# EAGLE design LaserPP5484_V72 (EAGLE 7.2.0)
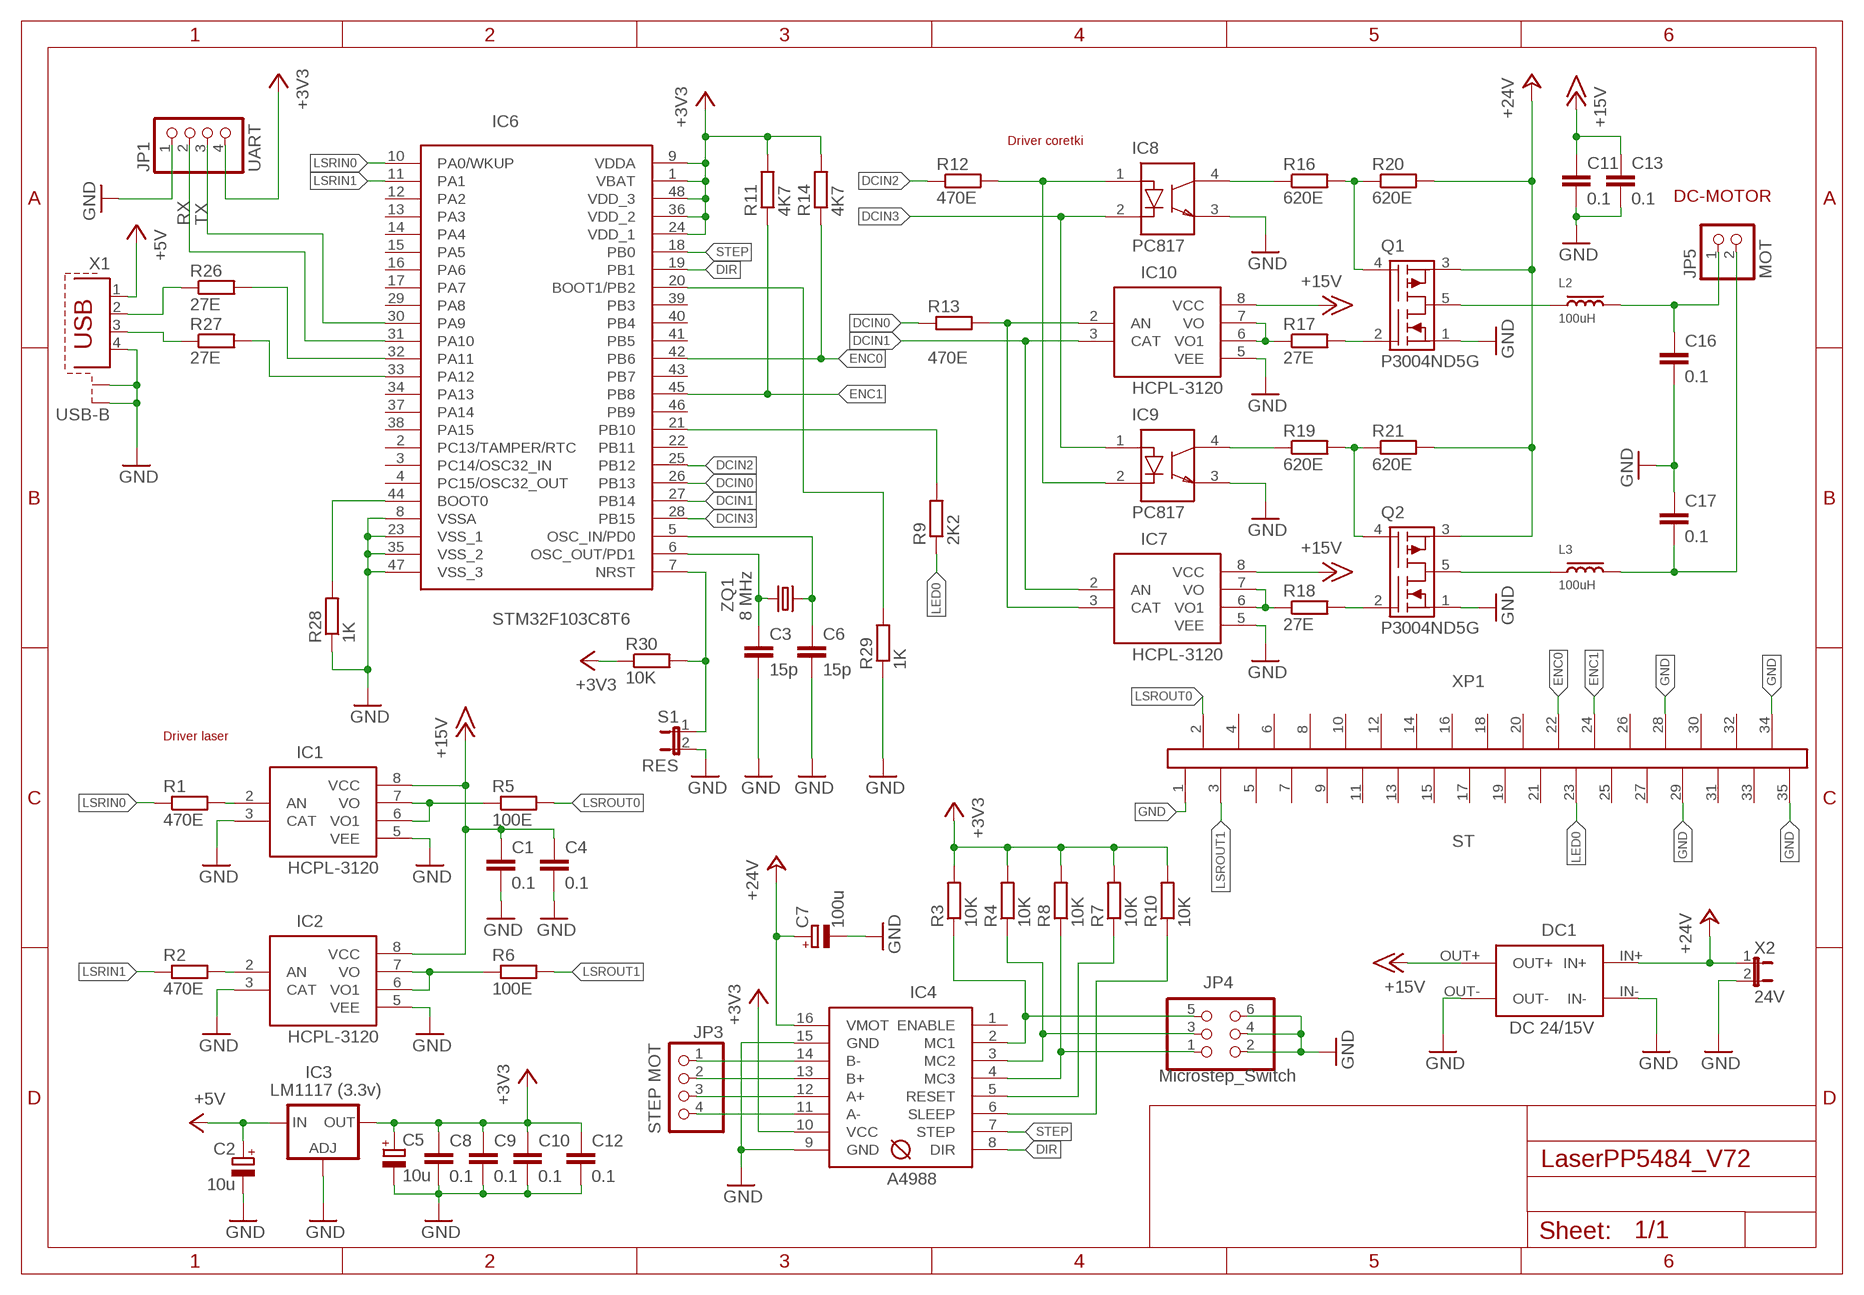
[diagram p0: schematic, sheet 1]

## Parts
C1  0.1  C-EUC0805  [C0805]
C2  10u  CPOL-EUSMCC  [SMC_C]
C3  15p  C-EUC0805  [C0805]
C4  0.1  C-EUC0805  [C0805]
C5  10u  CPOL-EUSMCA  [SMC_A]
C6  15p  C-EUC0805  [C0805]
C7  100u  CPOL-EUE2.5-7  [E2,5-7]
C8  0.1  C-EUC0805  [C0805]
C9  0.1  C-EUC0805  [C0805]
C10  0.1  C-EUC0805  [C0805]
C11  0.1  C-EUC0805  [C0805]
C12  0.1  C-EUC0805  [C0805]
C13  0.1  C-EUC0805  [C0805]
C16  0.1  C-EUC0805  [C0805]
C17  0.1  C-EUC0805  [C0805]
DC1  DC 24/15V  DC  [DC]
IC1  HCPL-3120  HCPL-3120DILSMD  [DIL08SMD]
IC2  HCPL-3120  HCPL-3120DILSMD  [DIL08SMD]
IC3  LM1117 (3.3v)  LM317MBSTT3  [SOT223]
IC4  A4988  [A4988]
IC6  STM32F103C8T6  STM32F100C4T  [LQFP48-7X7]
IC7  HCPL-3120  HCPL-3120DILSMD  [DIL08SMD]
IC8  PC817  [DIL04]
IC9  PC817  [DIL04]
IC10  HCPL-3120  HCPL-3120DILSMD  [DIL08SMD]
JP1  UART  PINHD-1X4  [1X04]
JP3  STEP MOT  PINHD-1X4  [1X04]
JP4  Microstep_Switch  PINHD-2X3  [2X03]
JP5  MOT  PINHD-1X2PW10-2-M  [PW10-2-M]
L2  100uH  L  [5_08]
L3  100uH  L  [5_08]
Q1  P3004ND5G  [TO252-51]
Q2  P3004ND5G  [TO252-51]
R1  470E  R-EU_R0805  [R0805]
R2  470E  R-EU_R0805  [R0805]
R3  10K  R-EU_R0805  [R0805]
R4  10K  R-EU_R0805  [R0805]
R5  100E  R-EU_0617/22  [0617/22]
R6  100E  R-EU_0617/22  [0617/22]
R7  10K  R-EU_R0805  [R0805]
R8  10K  R-EU_R0805  [R0805]
R9  2K2  R-EU_R0805  [R0805]
R10  10K  R-EU_R0805  [R0805]
R11  4K7  R-EU_R0805  [R0805]
R12  470E  R-EU_R0805  [R0805]
R13  470E  R-EU_R0805  [R0805]
R14  4K7  R-EU_R0805  [R0805]
R16  620E  R-EU_R0805  [R0805]
R17  27E  R-EU_R1206  [R1206]
R18  27E  R-EU_R1206  [R1206]
R19  620E  R-EU_R0805  [R0805]
R20  620E  R-EU_R0805  [R0805]
R21  620E  R-EU_R0805  [R0805]
R26  27E  R-EU_R1206  [R1206]
R27  27E  R-EU_R1206  [R1206]
R28  1K  R-EU_R0805  [R0805]
R29  1K  R-EU_R0805  [R0805]
R30  10K  R-EU_R0805  [R0805]
S1  RES  JP1E  [JP1]
X1  USB-B  PN61729-S  [PN61729-S]
X2  24V  PWL  [PWL]
XP1  ST  [ST]
ZQ1  8 MHz  CRYSTALHC49S  [HC49/S]

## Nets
+3V3: C5.+ C8.1 C9.1 C10.1 C12.1 IC3.4(OUT) IC4.10(VCC) IC6.1(VBAT) IC6.9(VDDA) IC6.24(VDD_1) IC6.36(VDD_2) IC6.48(VDD_3) JP1.4 R3.2 R4.2 R7.2 R8.2 R10.2 R11.2 R14.2 R30.1
+5V: C2.+ IC3.3(IN) X1.1
+15V: C1.1 C4.1 C11.1 C13.1 DC1.OUT+ IC1.8(VCC) IC2.8(VCC) IC7.8(VCC) IC10.8(VCC)
+24V: C7.+ DC1.IN+ IC4.16(VMOT) Q1.3(S2) Q2.3(S2) R20.2 R21.2 X2.1
DCIN0: IC6.26(PB13) R13.1
DCIN1: IC6.27(PB14) IC7.2(AN) IC10.3(CAT)
DCIN2: IC6.25(PB12) R12.1
DCIN3: IC6.28(PB15) IC8.2(K) IC9.1(A)
DIR: IC4.8(DIR) IC6.19(PB1)
ENC0: IC6.42(PB6) R14.1 XP1.22
ENC1: IC6.45(PB8) R11.1 XP1.24
GND: C1.2 C2.- C3.2 C4.2 C5.- C6.2 C7.- C8.2 C9.2 C10.2 C11.2 C12.2 C13.2 C16.2 C17.1 DC1.IN- DC1.OUT- IC1.3(CAT) IC1.5(VEE) IC2.3(CAT) IC2.5(VEE) IC3.1(ADJ) IC4.9(GND) IC4.15(GND) IC6.8(VSSA) IC6.23(VSS_1) IC6.35(VSS_2) IC6.47(VSS_3) IC7.5(VEE) IC8.3(E) IC9.3(E) IC10.5(VEE) JP1.1 JP4.2 JP4.4 JP4.6 Q1.1(S1) Q2.1(S1) R28.1 R29.1 S1.2 X1.4 X1.S1 X1.S2 X2.2 XP1.1 XP1.28 XP1.29 XP1.34 XP1.35
LED0: R9.1 XP1.23
LSRIN0: IC6.10(PA0/WKUP) R1.1
LSRIN1: IC6.11(PA1) R2.1
LSROUT0: R5.2 XP1.2
LSROUT1: R6.2 XP1.3
N$1: IC6.7(NRST) R30.2 S1.1
N$2: C3.1 IC6.6(OSC_OUT/PD1) ZQ1.1
N$3: C6.1 IC6.5(OSC_IN/PD0) ZQ1.2
N$4: R26.1 X1.2
N$5: IC6.32(PA11) R26.2
N$6: R27.1 X1.3
N$7: IC6.33(PA12) R27.2
N$8: IC4.11(A-) JP3.4
N$9: IC4.12(A+) JP3.3
N$10: IC1.2(AN) R1.2
N$11: IC4.13(B+) JP3.2
N$12: IC6.44(BOOT0) R28.2
N$14: IC2.2(AN) R2.2
N$15: IC6.21(PB10) R9.2
N$17: IC4.14(B-) JP3.1
N$18: IC4.2(MC1) JP4.5 R3.1
N$19: IC4.3(MC2) JP4.3 R4.1
N$20: IC4.4(MC3) JP4.1 R8.1
N$21: IC8.1(A) IC9.2(K) R12.2
N$22: IC8.4(C) R16.1
N$23: IC7.3(CAT) IC10.2(AN) R13.2
N$24: IC9.4(C) R19.1
N$25: IC10.6(VO1) IC10.7(VO) R17.1
N$26: IC7.6(VO1) IC7.7(VO) R18.1
N$27: Q1.2(G1) R17.2
N$28: L2.1 Q1.5(D1/D2)
N$29: Q1.4(G2) R16.2 R20.1
N$30: Q2.2(G1) R18.2
N$31: Q2.4(G2) R19.2 R21.1
N$32: L3.1 Q2.5(D1/D2)
N$33: C17.2 JP5.2 L3.2
N$34: C16.1 JP5.1 L2.2
N$35: IC4.5(RESET) R7.1
N$36: IC4.6(SLEEP) R10.1
N$39: IC1.6(VO1) IC1.7(VO) R5.1
N$41: IC2.6(VO1) IC2.7(VO) R6.1
N$48: IC6.20(BOOT1/PB2) R29.2
RX: IC6.31(PA10) JP1.2
STEP: IC4.7(STEP) IC6.18(PB0)
TX: IC6.30(PA9) JP1.3
Unconnected: IC4.1(ENABLE) IC6.2(PC13/TAMPER/RTC) IC6.3(PC14/OSC32_IN) IC6.4(PC15/OSC32_OUT) IC6.12(PA2) IC6.13(PA3) IC6.14(PA4) IC6.15(PA5) IC6.16(PA6) IC6.17(PA7) IC6.22(PB11) IC6.29(PA8) IC6.34(PA13) IC6.37(PA14) IC6.38(PA15) IC6.39(PB3) IC6.40(PB4) IC6.41(PB5) IC6.43(PB7) IC6.46(PB9) XP1.4 XP1.5 XP1.6 XP1.7 XP1.8 XP1.9 XP1.10 XP1.11 XP1.12 XP1.13 XP1.14 XP1.15 XP1.16 XP1.17 XP1.18 XP1.19 XP1.20 XP1.21 XP1.25 XP1.26 XP1.27 XP1.30 XP1.31 XP1.32 XP1.33

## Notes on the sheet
- Driver coretki
- DC-MOTOR
- Driver laser

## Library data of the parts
C1 C3 C4 C6 C8-C13 C16 C17 = rcl:C-EU: CAPACITOR, European symbol
C2 C5 C7 = rcl:CPOL-EU: POLARIZED CAPACITOR, European symbol
DC1 = LaserPP:DC
IC1 IC2 IC7 IC10 = LaserPP:HCPL-3120
IC3 = v-reg:LM317?*: 500 mA Adjustable Output Positive Voltage Regulator Source: http://www.onsemi.co.jp .. LM317M-D.PDF
IC4 = LaserPP:A4988
IC6 = Timer-stm32:STM32F100C4T
IC8 IC9 = LaserPP:PC817
JP1 JP3 = pinhead:PINHD-1X4: PIN HEADER
JP4 = LaserPP:PINHD-2X3: PIN HEADER
JP5 = BPPLS:PINHD-1X2: PIN HEADER
L2 L3 = LaserPP:L
Q1 Q2 = LaserPP:P3004ND5G
R1-R14 R16-R21 R26-R30 = rcl:R-EU_: RESISTOR, European symbol
S1 = jumper:JP1E: JUMPER
X1 = con-berg:PN61729-S: BERG USB connector
X2 = Timer-stm32:PWL
XP1 = LaserPP:ST
ZQ1 = crystal:CRYSTAL: CRYSTAL

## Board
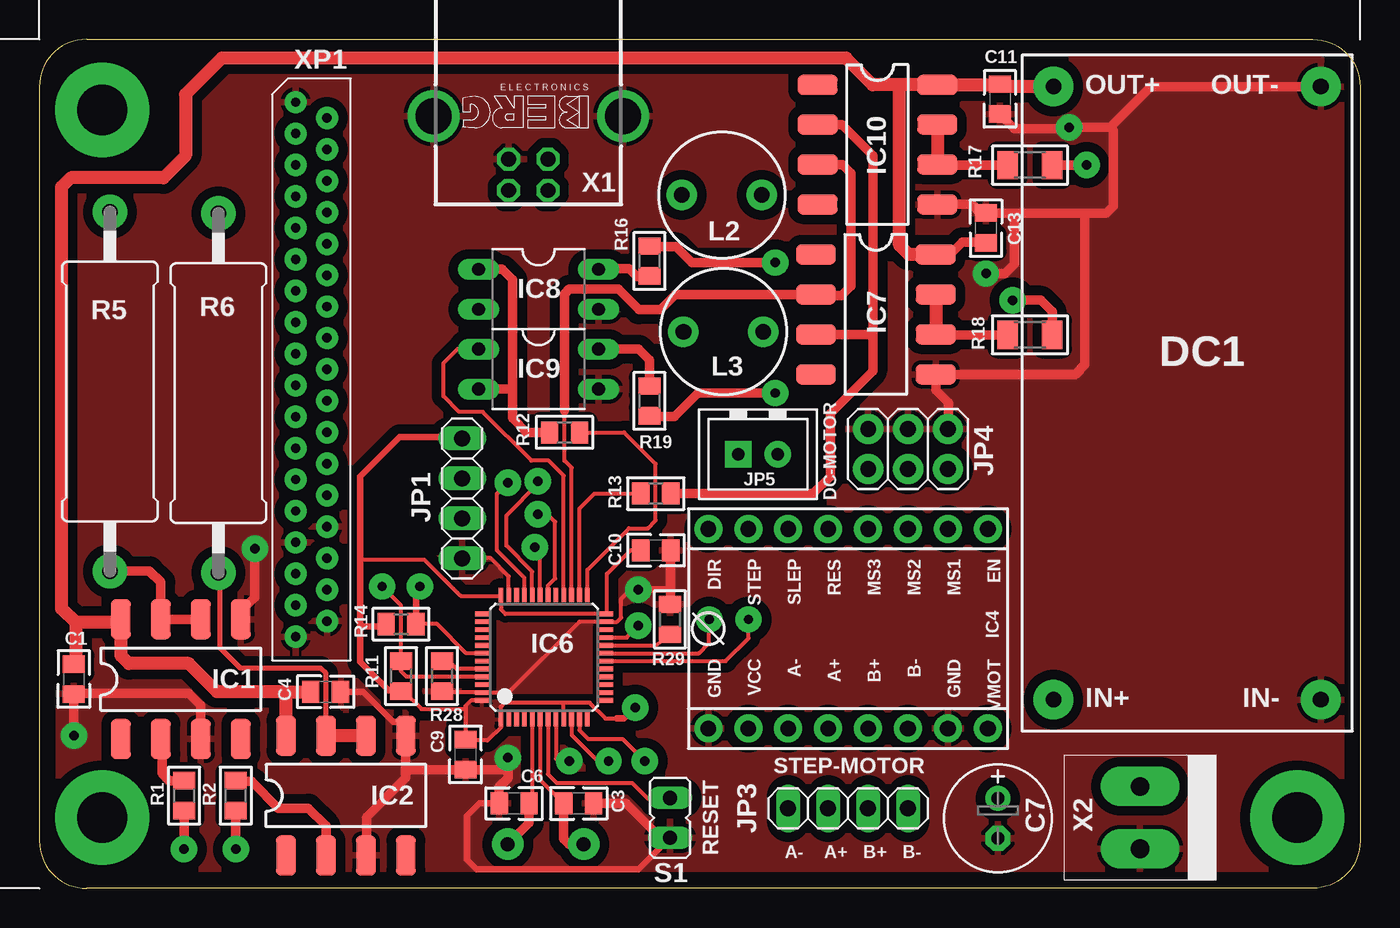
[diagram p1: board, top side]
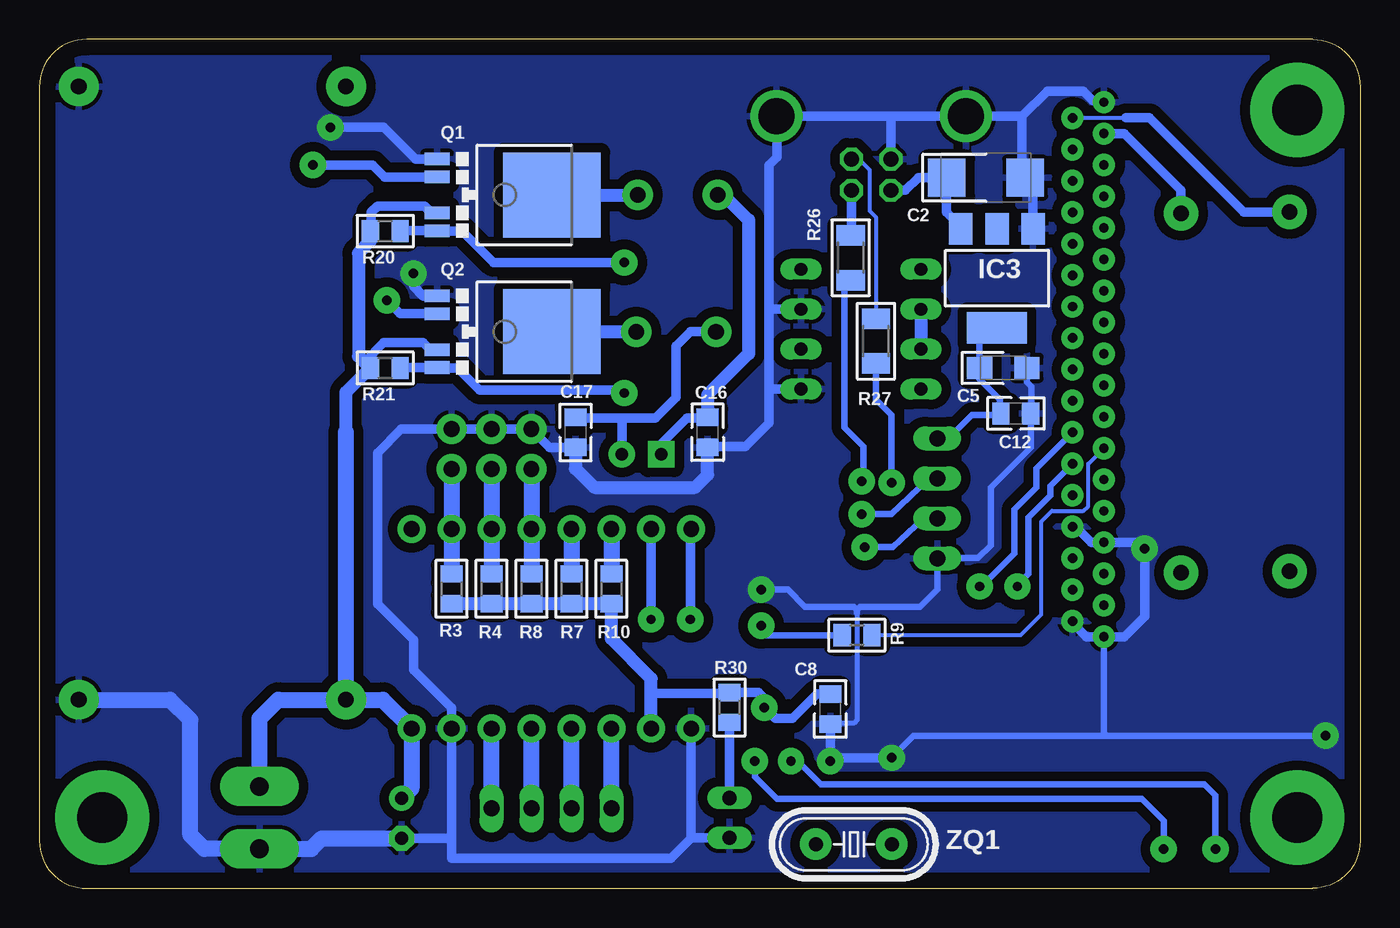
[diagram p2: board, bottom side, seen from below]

Size 84 x 54 mm. Coordinates in mm from the lower left corner, seen from the top.
Outline: 0,51 0,3 arc90 3,0 81,0 arc90 84,3 84,51 arc90 81,54 3,54 arc90 0,51
Copper layers (1*16): Top 0.035mm / dielectric 1.5mm / Bottom 0.035mm
Design rules "default *": minimum track width 10mil, minimum drill 24mil, track to track 8mil, track to pad 8mil, pad to pad 8mil, via to via 8mil, smd to smd 8mil, copper to edge 40mil, drill to drill 8mil, minimum pad ring 10mil, minimum via ring 8mil, stop-mask expansion 4mil, vias tented up to drill 0mil, thermal gap 10mil

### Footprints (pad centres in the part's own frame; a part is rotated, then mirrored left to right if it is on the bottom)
C0805 = smd 1.1 x 1.4: 1 -0.95,0; 2 0.95,0
SMC_C = smd 2.4 x 2.4: + -2.5,0; - 2.5,0
SMC_A = smd 1.6 x 1.4: + -1.5,0; - 1.5,0
E2,5-7 = drill 0.813 pad 1.6: + -1.27,0 | drill 0.813 pad 1.6 octagon: - 1.27,0
DC = drill 1 pad 2.54: IN+ 19.5,-8.5; IN- 19.5,8.5; OUT+ -19.5,-8.5; OUT- -19.5,8.5
DIL08SMD = smd 1.27 x 2.54: 1 -3.81,-3.81; 2 -1.27,-3.81; 3 1.27,-3.81; 4 3.81,-3.81; 5 3.81,3.81; 6 1.27,3.81; 7 -1.27,3.81; 8 -3.81,3.81
SOT223 = smd 1.5 x 2: 1 -2.3,-3.15; 2 0,-3.15; 3 2.3,-3.15 | smd 3.8 x 2: 4 0,3.15
A4988 = drill 1 pad 1.778: 1 -6.35,8.89; 2 -6.35,6.35; 3 -6.35,3.81; 4 -6.35,1.27; 5 -6.35,-1.27; 6 -6.35,-3.81; 7 -6.35,-6.35; 8 -6.35,-8.89; 9 6.35,-8.89; 10 6.35,-6.35; 11 6.35,-3.81; 12 6.35,-1.27; 13 6.35,1.27; 14 6.35,3.81; 15 6.35,6.35; 16 6.35,8.89
LQFP48-7X7 = smd 0.9 x 0.3: 1 -3.95,2.75; 2 -3.95,2.25; 3 -3.95,1.75; 4 -3.95,1.25; 5 -3.95,0.75; 6 -3.95,0.25; 7 -3.95,-0.25; 8 -3.95,-0.75; 9 -3.95,-1.25; 10 -3.95,-1.75; 11 -3.95,-2.25; 12 -3.95,-2.75; 25 3.95,-2.75; 26 3.95,-2.25; 27 3.95,-1.75; 28 3.95,-1.25; 29 3.95,-0.75; 30 3.95,-0.25; 31 3.95,0.25; 32 3.95,0.75; 33 3.95,1.25; 34 3.95,1.75; 35 3.95,2.25; 36 3.95,2.75 | smd 0.3 x 0.9: 13 -2.75,-3.95; 14 -2.25,-3.95; 15 -1.75,-3.95; 16 -1.25,-3.95; 17 -0.75,-3.95; 18 -0.25,-3.95; 19 0.25,-3.95; 20 0.75,-3.95; 21 1.25,-3.95; 22 1.75,-3.95; 23 2.25,-3.95; 24 2.75,-3.95; 37 2.75,3.95; 38 2.25,3.95; 39 1.75,3.95; 40 1.25,3.95; 41 0.75,3.95; 42 0.25,3.95; 43 -0.25,3.95; 44 -0.75,3.95; 45 -1.25,3.95; 46 -1.75,3.95; 47 -2.25,3.95; 48 -2.75,3.95
DIL04 = drill 0.813 long: 1 -1.27,-3.81; 2 1.27,-3.81; 3 1.27,3.81; 4 -1.27,3.81
1X04 = drill 1.016 long: 1 -3.81,0; 2 -1.27,0; 3 1.27,0; 4 3.81,0
2X03 = drill 1 pad 1.93: 1 -2.54,-1.27; 2 -2.54,1.27; 3 0,-1.27; 4 0,1.27; 5 2.54,-1.27; 6 2.54,1.27
PW10-2-M = drill 0.8 pad 1.676 square: 1 -1.25,0 | drill 0.8 pad 1.676: 2 1.25,0
5_08 = drill 1 pad 1.93: 1 -2.54,0; 2 2.54,0
TO252-51 = smd 0.8 x 1.6: 1 -2.28,-4.8; 2 -1.14,-4.8; 3 1.14,-4.8; 4 2.28,-4.8 | smd 5.4 x 6.2: 5 0,2.5
R0805 = smd 1.1 x 1.4: 1 -0.95,0; 2 0.95,0
0617/22 = drill 1 pad 2.184: 1 -11.43,0; 2 11.43,0
R1206 = smd 1.3 x 1.8: 1 -1.422,0; 2 1.422,0
JP1 = drill 0.914 long: 1 0,-1.27; 2 0,1.27
PN61729-S = drill 0.95 octagon: 1 1.25,4.71; 2 -1.25,4.71; 3 -1.25,2.71; 4 1.25,2.71 | drill 2.3 pad 2.9: S1 -6.02,0; S2 6.02,0
PWL = drill 1.2 pad 2.5 long: 1 -1.97,0; 2 1.99,0
ST = drill 0.6 pad 1.422: 1 -17,-1; 2 -16,1; 3 -15,-1; 4 -14,1; 5 -13,-1; 6 -12,1; 7 -11,-1; 8 -10,1; 9 -9,-1; 10 -8,1; 11 -7,-1; 12 -6,1; 13 -5,-1; 14 -4,1; 15 -3,-1; 16 -2,1; 17 -1,-1; 18 0,1; 19 1,-1; 20 2,1; 21 3,-1; 22 4,1; 23 5,-1; 24 6,1; 25 7,-1; 26 8,1; 27 9,-1; 28 10,1; 29 11,-1; 30 12,1; 31 13,-1; 32 14,1; 33 15,-1; 34 16,1; 35 17,-1
HC49/S = drill 0.9 pad 2: 1 -2.413,0; 2 2.413,0

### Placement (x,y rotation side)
C1  2.2,13.3 270 top
C2  23.8,45.2 0 bottom
C3  34.3,5.4 0 top
C4  18.2,12.5 0 top
C5  22.7,33.1 0 bottom
C6  30.2,5.4 180 top
C7  60.96,4.45 270 top
C8  33.7,11.4 270 bottom
C9  27.1,8.5 270 top
C10  39.2,21.5 0 top
C11  61.1,50.2 270 top
C12  21.9,30.2 0 bottom
C13  60.2,42 90 top
C16  41.5,29 270 bottom
C17  49.9,29 90 bottom
DC1  73,31.5 270 top
IC1  9,13.3 0 top
IC2  19.5,5.9 0 top
IC3  23.1,38.8 180 bottom
IC4  51.44,16.51 270 top
IC6  32.1,14.7 90 top
IC7  53.2,36.5 270 top
IC8  31.75,38.1 270 top
IC9  31.75,33.02 270 top
IC10  53.3,47.3 270 top
JP1  26.9,24.8 90 top
JP3  51.44,5.08 180 top
JP4  55.24,27.94 0 top
JP5  45.7,27.6 0 top
L2  43.4,44.1 180 top
L3  43.5,35.4 180 top
Q1  53.9,44.1 270 bottom
Q2  53.9,35.4 270 bottom
R1  9.2,5.9 90 top
R2  12.5,5.9 90 top
R3  57.78,19.05 270 bottom
R4  55.24,19.05 270 bottom
R5  4.49,31.6 90 top
R6  11.39,31.5 90 top
R7  50.16,19.05 270 bottom
R8  52.7,19.05 270 bottom
R9  32,16.1 180 bottom
R10  47.62,19.05 270 bottom
R11  23,13.5 270 top
R12  33.4,29 180 top
R13  39.2,25.1 0 top
R14  23,16.8 180 top
R16  38.8,39.9 90 top
R17  63,46 0 top
R18  63,35.2 0 top
R19  38.8,31 270 top
R20  62,41.8 180 bottom
R21  62,33.1 180 bottom
R26  32.4,40.1 270 bottom
R27  30.8,34.8 270 bottom
R28  25.6,13.5 90 top
R29  40.1,17.1 270 top
R30  40.1,11.5 270 bottom
S1  40.11,4.48 180 top
X1  31.1,49.1 180 top
X2  70,4.5 270 top
XP1  17.3,33 270 top
ZQ1  32.2,2.8 0 bottom

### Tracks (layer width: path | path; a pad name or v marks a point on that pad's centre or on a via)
+3V3  (via drill 0.6 pad 1.68)
  Top 0.254: 33.3,11.8 35,11.8 36,10.8 36.7,10.8 | 33.3,11.8 29.6,11.8 29.35,11.55 IC6.1 29.35,10.25 28.5,9.4 27.15,9.4 C9.1 27.1,11.4 | IC6.9 33.35,11.75 33.3,11.8 | IC6.48 27.45,11.95 27.1,11.6 27.1,11.4 | R11.2 23.15,12.55 24.3,11.4 27.1,11.4 | 20.4,21 20.5,20.9 24.5,20.9 26.8,18.6 29.3,18.6 IC6.36 29.35,17.75 29.65,17.45 IC6.24 36.1,17.5 36.1,20 37.6,21.5 C10.1
  Top 0.406: 36.7,10.8 37.2,10.8 v37.9,11.5 | R14.2 22.05,16.65 20.45,16.65 20.4,16.7 | R11.2 22.95,12.6 22.2,12.6 20.4,14.4 20.4,16.7 | 20.4,16.7 20.4,21 20.4,26.2 22.9,28.7 26.81,28.7 JP1.4
  Bottom 0.406: IC3.4 23.35,35.65 24.2,34.8 C5.+ 24.2,32.4 22.9,31.1 22.9,30.25 C12.1 22.95,30.1 24.7,30.1 26.19,28.61 JP1.4
  Bottom 0.61: 45.09,12.4 40.15,12.4 R30.1 38.25,12.45 37.9,12.1 v37.9,11.5 37.2,10.8 36.1,10.8 34.55,12.35 C8.1
  Bottom 0.813: IC4.10 45.09,12.4 45.09,13.34 47.62,15.88 R10.2 R7.2 R8.2 R4.2 R3.2
  pour Top: 27.4,11.9 29,11.9 29.3,11.6 29.3,10.2 28.5,9.4 27.3,9.4 27.1,9.6 27.1,11.6
+5V
  Bottom 0.61: X1.1 28.91,44.39 28.1,45.2 C2.+ 26.3,43 25.4,42.1 IC3.3
+15V
  Top 0.61: IC7.8 57.91,40.31 58.7,41.1 60.15,41.1 C13.1
  Top 0.813: 61.15,51.2 C11.1 | C11.1 61.06,51.11 IC10.8 54.7,51.11 | 54.7,51.11 52.99,51.11 51.3,52.8 11.6,52.8 9.3,50.5 9.3,46.6 7.9,45.2 2,45.2 1.4,44.6 1.4,17.8 2.3,16.9 | IC7.8 55.29,40.31 54.7,40.9 54.7,51.11 | 2.3,16.9 2.3,14.35 C1.1 | 2.3,16.9 5,16.9 5.19,17.09 IC1.8 5.19,14.81 5.7,14.3 9.5,14.3 11.3,12.5 15.7,12.5 | 15.7,12.5 C4.1 | IC2.8 15.69,12.49 15.7,12.5 | DC1.OUT+ 61.25,51 C11.1
+24V
  Bottom 0.61: Q2.3 59.16,34.26 59.6,34.7 62.1,34.7 63.33,33.48 | Q1.3 59.06,42.96 59.5,43.4 62.5,43.4 62.9,43 62.9,41.85 R20.2
  Bottom 0.813: R21.2 62.95,32.85 | R20.2 62.95,41.15 63.7,40.4 63.7,33.85 63.33,33.48 R21.2 | 64.5,29 64.5,31.55 R21.2
  Bottom 1.016: X2.1 70,10.8 68.8,12 DC1.IN+ | C7.+ 60.33,6.35 IC4.16 62.16,12 DC1.IN+ | DC1.IN+ 64.5,29
DCIN0
  Top 0.254: IC6.26 34.35,24.15 35.3,25.1 R13.1
DCIN1
  Top 0.254: 33.4,30.4 33.4,27.2 33.85,26.75 IC6.27
  Top 0.61: IC10.3 51.07,46.03 51.6,45.5 51.6,38.3 51,37.7 49.46,37.7 IC7.2 40.47,37.77 39.5,36.8 38.13,36.8 36.83,38.1 33.7,38.1 33.4,37.8 33.4,30.4
DCIN2
  Top 0.254: R12.1 37.2,29 39.2,27 39.2,23.4 38.7,22.9 37.5,22.9 34.85,20.25 IC6.25
DCIN3
  Top 0.254: IC6.28 33.35,26.25 32.4,27.2 31.3,27.2 28.2,30.3 26.7,30.3 25.7,31.3 25.7,33.4 26.6,34.3 IC9.1
  Bottom 0.813: IC8.2 IC9.1
DIR  (via drill 0.6 pad 1.68)
  Top 0.254: IC6.19 41.95,14.95 42.6,15.6 v42.6,17.1
  Bottom 0.61: v42.6,17.1 42.6,22.8 IC4.8
ENC0  (via drill 0.6 pad 1.68)
  Top 0.254: IC6.42 27.15,14.95 25.3,16.8 R14.1
  Top 0.406: R14.1 23.95,18.95 v24.2,19.2
  Bottom 0.406: v24.2,19.2 24.1,19.2 22,21.3 22,24.1 20.6,25.5 20.6,26.7 XP1.22
ENC1  (via drill 0.6 pad 1.68)
  Top 0.254: IC6.45 23.35,13.45 23,13.8 R11.1 23,18 v21.8,19.2
  Bottom 0.406: v21.8,19.2 21.8,19.3 21.1,20 21.1,23.6 19.7,25 19.7,25.6 XP1.24
GND  (via drill 0.6 pad 1.68)
  Top 0.254: IC6.8 32.85,8.25 33,8.1 v33.7,8.1 | R28.1 25.7,12.45 IC6.47 29.85,12.45 34.35,16.95 IC6.23 36.75,16.95 37,17.2 37,18.4 37.6,19 v38.1,19 | 40.05,18 R29.1 | IC6.35 29.85,19.85 28.7,21 JP1.1
  Top 0.406: S1.2 38.1,1.2 27.8,1.2 27.2,1.8 27.2,4.6 28,5.4 C6.2 | C4.2 20.6,12.5 22.5,10.6 23.1,10.6 23.3,10.4 IC2.5 | v38.1,19 40.15,19
  Top 0.61: 62.1,42.95 C13.2 59.85,42.95 59.3,43.5 IC10.5 | 62.1,42.95 66.5,42.95 | v60.2,39.1 61.4,39.1 62,39.7 62,42.85 62.1,42.95 | JP4.6 57.8,29.23 57.8,30.9 57.01,31.69 IC7.5 65.89,32.69 66.5,33.3 66.5,42.95 | S1.2 39.49,3.21 37.3,5.4 C3.2 | C6.2 29.25,6.45 29.8,7 29.8,7.8 | 29.8,7.8 v29.8,8.3 | 29.8,7.8 29.55,7.55 C9.2 23.36,7.55 23.31,7.6 | IC2.5 23.31,7.6 | 23.31,7.6 23.31,7.01 20.8,4.5 20.8,2.12 IC2.3 | IC1.3 10.27,11.63 9.5,12.4 2.25,12.4 C1.2 v2.2,9.7 | v13.7,21.6 13.7,18.5 12.9,17.7 12.9,17.2 IC1.5 | C10.2 40.15,19 40.15,18.1 R29.1 | C11.2 61.1,49.2 62,48.3 65.4,48.3 v65.5,48.4 68.1,48.4 | DC1.OUT- 70.7,51 68.1,48.4 | 66.5,42.95 67.85,42.95 68.3,43.4 68.3,48.2 68.1,48.4
  Bottom 0.305: 32,17.5 32,10.7 32.2,10.5 33.65,10.5 C8.2
  Bottom 0.406: v2.2,9.7 16.1,9.7 | 16.1,9.7 28.4,9.7 v29.8,8.3 | XP1.35 16.3,9.9 16.1,9.7 | C5.- 21.2,32.2 20.9,31.9 20.9,30.25 C12.2 20.95,28.05 23.5,25.5 23.5,21.8 24.3,21 JP1.1 26.9,19 28,17.9 31.8,17.9 32,17.7 | 32,17.7 32,17.5 | v38.1,19 36.4,19 35.3,17.9 32.2,17.9 32,17.7
  Bottom 0.61: IC4.9 42.55,3.17 | 42.55,3.17 43.81,1.91 57.78,1.91 57.78,3.17 | 57.78,3.17 IC4.15 57.78,11.48 60.2,13.9 60.2,15.8 62.5,18.1 62.5,27.7 61,29.2 57.8,29.2 JP4.6 JP4.4 JP4.2 51.55,28.05 C17.1 | C7.- 57.78,3.17 | Q1.1 60.08,46.38 62.1,48.4 v65.5,48.4 | Q2.1 59.58,37.68 60.2,38.3 v60.2,39.1 | S1.2 42.51,3.21 42.55,3.17 | C8.2 v33.7,8.1 33.5,8.3 v29.8,8.3 | XP1.1 17,50.1 17.6,50.7 19.9,50.7 21.5,49.1 | 21.5,49.1 X1.S2 29.9,49.1 | 29.9,49.1 X1.S1 37.1,49.08 37.1,46.5 37.6,46 37.6,36.8 | X1.4 29.85,49.05 29.9,49.1 | 37.6,31.7 37.6,29.6 39.1,28.1 41.45,28.1 C16.2 | 37.6,31.7 37.6,36.8 | IC8.3 37.57,36.83 37.6,36.8 | IC9.3 37.55,31.75 37.6,31.7 | IC3.1 20.8,44.7 C2.- 21.3,46.1 21.5,46.3 21.5,49.1 | XP1.34 18.3,16.9 17.4,16 XP1.35 15,16 13.7,17.3 v13.7,21.6 13.9,21.6 14.3,22 XP1.29 17.1,22 18.1,23 XP1.28
  Bottom 0.813: C17.1 49.9,26.7 48.7,25.5 42.3,25.5 41.5,26.3 C16.2
  Bottom 1.016: C7.- 66.04,3.17 66.7,2.51 X2.2 73.51,2.51 74.4,3.4 74.4,10.7 75.7,12 DC1.IN-
  pour Bottom (isolate 0.61): 0,51 0,3 arc90 3,0 82,0 arc90 84,3 84,51 arc90 81,54 3,54 arc90
  pour Top (isolate 0.61): 0,51 0,3 arc90 3,0 81,0 arc90 84,3 84,51 arc90 81,54 3,54 arc90
  pour Top (isolate 0.406): 29.2,17 29.2,12.5 35.1,12.3 35.1,17
LED0
  Bottom 0.254: R9.1 21.6,16.1 20.3,17.4 20.3,23.3 19.6,24 17.6,24 17.3,24.3 17.3,27 XP1.23
LSRIN0  (via drill 0.6 pad 1.68)
  Top 0.254: IC6.10 33.85,9.75 35.5,8.1 v36.2,8.1
  Top 0.61: R1.1 v9.2,2.5
  Bottom 0.406: v36.2,8.1 35.8,8.1 34.3,6.6 9.9,6.6 9.2,5.9 v9.2,2.5
LSRIN1  (via drill 0.6 pad 1.68)
  Top 0.254: IC6.11 34.35,10.05 34.9,9.5 37.1,9.5 v38.5,8.1
  Top 0.61: R2.1 v12.5,2.5
  Bottom 0.406: v12.5,2.5 12.5,4.3 13.9,5.7 37.1,5.7 38.5,7.1 v38.5,8.1
LSROUT0
  Bottom 0.254: XP1.2 14.9,49
  Bottom 0.61: 14.9,49 13.4,49 7.4,43 4.52,43 R5.2
LSROUT1
  Bottom 0.61: XP1.3 15,48 11.4,44.4 R6.2
N$1
  Top 0.254: IC6.7 32.35,7.25 32.9,6.7 37.7,6.7 38.7,5.7 40.06,5.7 S1.1
  Bottom 0.61: R30.2 S1.1
N$2
  Top 0.254: IC6.6 31.85,6.9 C3.1
  Top 0.61: C3.1 33.35,3.15 33.7,2.8 ZQ1.1
N$3
  Top 0.254: IC6.5 31.35,5.6 C6.1
  Top 0.61: C6.1 31.15,4.16 ZQ1.2
N$4
  Bottom 0.61: X1.2 32.35,41.57 R26.1
N$5  (via drill 0.6 pad 1.68)
  Top 0.254: v31.7,25.9 31.7,25.7 29.7,23.7 29.7,21.8 31.35,20.15 IC6.32
  Bottom 0.406: R26.2 32.4,38.6 32.8,38.2 32.8,29.3 31.6,28.1 31.6,26 v31.7,25.9
N$6
  Bottom 0.254: X1.3 31.89,46.39 31.2,45.7 31.2,43.1 30.8,42.7 R27.1
N$7  (via drill 0.6 pad 1.68)
  Top 0.254: IC6.33 30.85,19.75 29.1,21.5 29.1,25.1 v29.8,25.8
  Bottom 0.406: v29.8,25.8 29.8,30.1 30.8,31.1 R27.2
N$8
  Bottom 1.016: JP3.4 IC4.11
N$9
  Bottom 1.016: JP3.3 IC4.12
N$10
  Top 0.61: R1.2 8.25,6.85 7.8,7.3 7.8,9.42 IC1.2
N$11
  Bottom 1.016: JP3.2 IC4.13
N$12
  Top 0.254: IC6.44 26.55,13.95 26.1,14.4 25.65,14.4 R28.2
N$14
  Top 0.61: R2.2 12.55,6.8 13.5,6.8 15.2,5.1 17.1,5.1 18.23,3.97 IC2.2
N$15  (via drill 0.6 pad 1.68)
  Top 0.254: IC6.21 37.35,15.95 v38.1,16.7
  Bottom 0.406: v38.1,16.7 38.1,16.3 37.9,16.1 R9.2
N$17
  Bottom 1.016: JP3.1 IC4.14
N$18
  Bottom 1.016: JP4.5 IC4.2 R3.1
N$19
  Bottom 1.016: JP4.3 IC4.3 R4.1
N$20
  Bottom 1.016: JP4.1 IC4.4 R8.1
N$21
  Top 0.61: IC8.1 29.43,39.37 30.1,38.7 30.1,31.7 | 30.1,31.7 30.1,29.9 31,29 R12.2 | IC9.2 30.05,31.75 30.1,31.7
N$22
  Top 0.61: R16.1 38.75,38.9 38,38.9 37.5,39.4 35.59,39.4 IC8.4
N$23
  Top 0.61: IC10.2 51.03,48.57 53,46.6 53,35.2 | 53,35.2 53,32.9 50.3,30.2 50.3,26.2 49.2,25.1 R13.2 | IC7.3 52.97,35.23 53,35.2
N$24
  Top 0.61: IC9.4 38.11,34.29 38.8,33.6 R19.1
N$25
  Top 0.61: R17.1 57.11,46 IC10.6
  Top 0.813: IC10.7 IC10.6
N$26
  Top 0.61: R18.1 57.01,35.2 IC7.6
  Top 0.813: IC7.7 IC7.6
N$27  (via drill 0.6 pad 1.68)
  Top 0.61: R17.2 v66.6,46
  Bottom 0.61: Q1.2 62.04,45.24 62.8,46 v66.6,46
N$28
  Bottom 0.813: Q1.5 L2.1
N$29  (via drill 0.6 pad 1.68)
  Top 0.61: v46.8,39.8 41.5,39.8 40.5,40.8 38.85,40.8 R16.2
  Bottom 0.61: R20.1 61.03,41.82 Q1.4 58.68,41.8 57.1,41.8 55.1,39.8 v46.8,39.8
N$30  (via drill 0.6 pad 1.68)
  Top 0.61: R18.2 64.42,36.68 63.7,37.4 v61.9,37.4
  Bottom 0.61: Q2.2 61.04,36.54 v61.9,37.4
N$31  (via drill 0.6 pad 1.68)
  Top 0.61: v46.8,31.5 41.9,31.5 40.4,30 38.85,30 R19.2
  Bottom 0.61: R21.1 61.03,33.12 Q2.4 58.68,33.1 57.4,33.1 56,31.7 47,31.7 v46.8,31.5
N$32
  Bottom 0.813: Q2.5 L3.1
N$33
  Bottom 0.61: L3.2 42.6,35.4 43.5,34.5 43.5,31.2 44.8,29.9 46.9,29.9 | 49.85,29.9 46.9,29.9 | JP5.2 46.95,29.85 46.9,29.9
  Bottom 0.813: 49.85,29.9 C17.2
N$34
  Bottom 0.61: JP5.1 44.45,28.25 42.8,29.9 41.55,29.9
  Bottom 0.813: L2.2 40.5,44.1 38.9,42.5 38.9,34 41.5,31.4 C16.1 41.55,29.9
N$35
  Bottom 1.016: IC4.5 R7.1
N$36
  Bottom 1.016: IC4.6 R10.1
N$37  (via drill 3.2 pad 6)
  other vias: 80,4.5
N$38  (via drill 3.2 pad 6)
  other vias: 4,4.5
N$39
  Top 0.61: IC1.6 IC1.7 7.73,19.47 7,20.2 4.52,20.2 R5.1
N$40  (via drill 3.2 pad 6)
  other vias: 4,49.5
N$41
  Top 0.305: IC2.7 18.23,13.67 17.9,14 12.8,14 11.5,15.3 11.5,19.96 R6.1
  Top 0.813: IC2.6 IC2.7
N$48
  Top 0.254: IC6.20 39.2,15.45 R29.2
RX  (via drill 0.6 pad 1.68)
  Top 0.254: IC6.31 31.85,21.45 v31.5,21.7
  Bottom 0.406: JP1.2 26.93,23.5 27.8,23.5 29.7,21.7 v31.5,21.7
STEP  (via drill 0.6 pad 1.68)
  Top 0.254: IC6.18 43.65,14.45 45.1,15.9 v45.1,17.1
  Bottom 0.61: v45.1,17.1 45.1,22.84 IC4.7
TX  (via drill 0.6 pad 1.68)
  Top 0.254: IC6.30 32.35,19.25 32.8,19.7 32.8,23.3 32.3,23.8 v31.7,23.8
  Bottom 0.406: JP1.3 26.97,26 27.5,26 29.8,23.8 v31.7,23.8

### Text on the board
tPlace: DC-MOTOR | STEP-MOTOR | RESET | A- | A+ | B+ | B-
